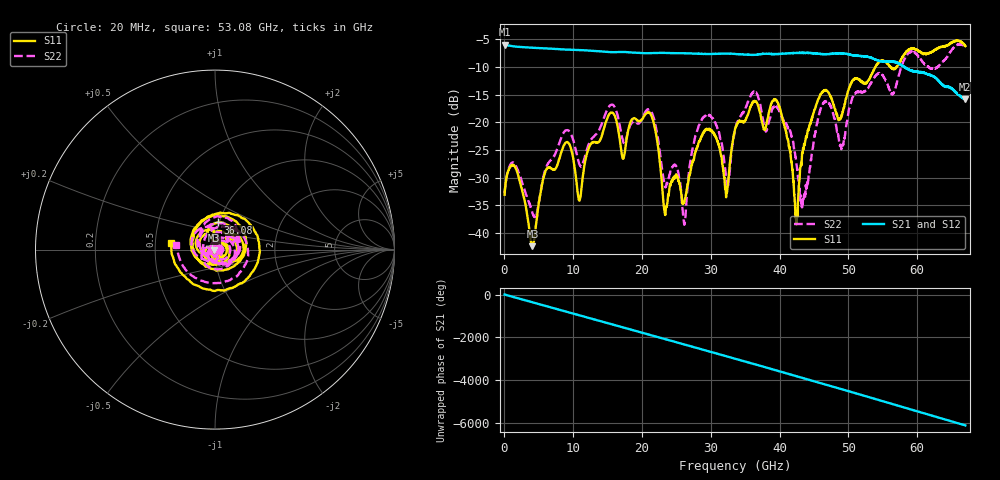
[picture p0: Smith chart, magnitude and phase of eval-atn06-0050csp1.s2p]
!Keysight Technologies,N5247B,US58420632,A.14.00.23
!Date: Monday, April 25, 2022 11:30:59
!Correction: S11(C  2-Port  )
!S21(C  2-Port  )
!S12(C  2-Port  )
!S22(C  2-Port  )
!S2P File: Measurement: :
# Hz S  dB  R 50
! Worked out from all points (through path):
!   3350 points, 20 MHz to 67 GHz, reference 50 ohm
!   highest |S21| = -6.00 dB at 20 MHz (marker M1); lowest = -15.9 dB at 66.96 GHz (marker M2)
!   group delay of S21, straight-line fit = 252 ps
!   lowest |S11| = -42.3 dB at 4.06 GHz (marker M3), VSWR 1.02, Z = 49.3 - j0.378 ohm
!   |S11| at or under -10 dB: start of sweep to 53.9 GHz; 56.06 GHz to 57.01 GHz (958.4 MHz wide, 1.7 % of centre)
!   |S22| runs from -38.5 to -5.9 dB; largest |S21 - S12| = 0.0037
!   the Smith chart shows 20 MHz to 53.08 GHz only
!   S11 on the Smith chart (normalised r, x): 20 MHz: 1.05, +0.00; 36.08 GHz: 0.98, +0.30; 53.08 GHz: 0.60, +0.05
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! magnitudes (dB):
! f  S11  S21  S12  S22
! 20 MHz  -33.1  -6.0  -6.0  -32.8
! 1.6 GHz  -28.2  -6.3  -6.3  -27.7
! 4.06 GHz  -42.3  -6.5  -6.6  -36.3
! 8.84 GHz  -23.7  -6.9  -6.9  -21.5
! 11.2 GHz  -31.8  -7.0  -7.0  -27.9
! 15.46 GHz  -18.3  -7.3  -7.3  -16.9
! 22.36 GHz  -24.7  -7.5  -7.5  -23.3
! 23.34 GHz  -36.6  -7.5  -7.5  -31.6
! 26.1 GHz  -34.6  -7.5  -7.5  -38.3
! 28.68 GHz  -22.5  -7.6  -7.7  -19.4
! 32.26 GHz  -32.8  -7.6  -7.6  -30.8
! 33.52 GHz  -21.1  -7.7  -7.7  -21.4
! 36.08 GHz  -16.4  -7.8  -7.8  -14.6
! 39.8 GHz  -16.7  -7.7  -7.7  -17.5
! 42.42 GHz  -37.0  -7.5  -7.5  -27.2
! 43.4 GHz  -24.6  -7.4  -7.5  -34.0
! 44.68 GHz  -19.3  -7.5  -7.5  -25.5
! 46.42 GHz  -14.3  -7.7  -7.7  -16.5
! 53.08 GHz  -12.0  -8.3  -8.3  -13.3
! 55.84 GHz  -9.6  -9.0  -9.0  -13.6
! 66.96 GHz  -6.2  -15.9  -15.9  -6.3
! 67 GHz  -6.2  -15.9  -15.9  -6.4
